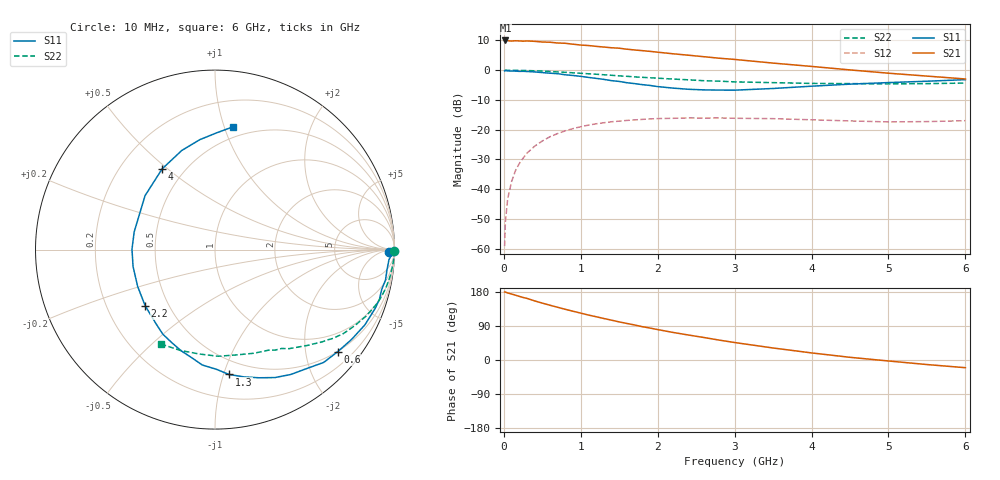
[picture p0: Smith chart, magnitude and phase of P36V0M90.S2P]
! SIEMENS Small Signal Semiconductors
! BFP181
! Si NPN RF Bipolar Junction Transistor in SOT143
! VCE = 6 V  IC = 0.9 mA
! Common Emitter S-Parameters:  March  1996
# GHz  S  MA  R  50
!  f  S11  S21  S12  S22
! GHz  MAG  ANG  MAG  ANG  MAG  ANG  MAG  ANG
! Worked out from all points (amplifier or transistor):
!   36 points, 10 MHz to 6 GHz, reference 50 ohm
!   highest |S21| = 10.0 dB at 20 MHz (marker M1)
!   |S21| within 3 dB of that: start of sweep to 1.624 GHz
!   unconditionally stable (mu >= 1): 3.315 GHz to end of sweep
!   at 250 MHz: K = 0.08, MSG = 19.7 dB, |S12| = -29.6 dB
!   at 1.4 GHz: K = 0.47, MSG = 12.4 dB, |S12| = -17.3 dB
!   at 6 GHz: K = 1.29, MAG = 3.8 dB, |S12| = -17.0 dB
!   S11 on the Smith chart (normalised r, x): 10 MHz: 50, -24; 600 MHz: 0.49, -2.68; 1.3 GHz: 0.38, -1.04; 2.2 GHz: 0.37, -0.31; 4 GHz: 0.38, +0.48; 6 GHz: 0.41, +1.07
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0.01  0.9678 -0.9  3.105 179.5  0.0011 79.7  0.9982 -0.3
0.02  0.9848 -1.6  3.158 179.3  0.0028 89.9  0.9975 -0.6
0.05  0.9709 -3.3  3.127 177.0  0.0069 87.7  0.9962 -1.6
0.1  0.9649 -6.7  3.085 174.1  0.0133 83.9  0.9969 -3.2
0.15  0.9651 -10.1  3.119 171.1  0.0203 82.2  0.9944 -4.8
0.3  0.9505 -20.2  3.099 162.6  0.0402 77.3  0.9846 -9.5
0.4  0.9344 -26.7  3.052 156.0  0.0527 72.1  0.9761 -12.6
0.6  0.8893 -39.8  2.949 144.5  0.0761 63.5  0.9516 -18.4
0.8  0.8358 -52.6  2.83 133.7  0.0956 55.5  0.92 -23.7
1.1  0.7553 -71.0  2.595 118.6  0.1192 44.9  0.8697 -30.9
1.3  0.7001 -83.6  2.447 109.5  0.1306 38.4  0.8368 -35.2
1.5  0.6468 -96.3  2.338 100.5  0.1391 32.8  0.8015 -39.0
1.8  0.5707 -115.2  2.129 87.9  0.1489 25.9  0.7585 -43.9
2.2  0.4992 -141.2  1.885 72.7  0.1552 17.5  0.7081 -50.3
2.4  0.4774 -154.5  1.784 65.9  0.1574 13.8  0.6886 -53.3
2.8  0.4626 179.8  1.588 52.5  0.1575 7.9  0.6534 -58.9
3  0.461 167.6  1.515 46.1  0.1554 5.4  0.6355 -61.8
3.5  0.4921 142.4  1.315 31.7  0.1531 0.6  0.6168 -69.4
4  0.5377 123.2  1.156 18.7  0.1465 -2.6  0.599 -78.4
4.5  0.5822 108.6  1.01 7.1  0.1402 -4.9  0.5944 -88.3
5.5  0.6519 88.9  0.795 -12.0  0.1366 -1.5  0.5941 -109.1
6  0.6925 81.5  0.711 -20.3  0.1415 -0.3  0.6066 -119.9
